FUNCTION p11_logicnaFunkcija : BOOL
VAR_INPUT
	x1: BOOL;
	x2: BOOL;
END_VAR
VAR_OUTPUT
	y: BOOL;
END_VAR
VAR // added by the converter: edge detectors and wires of the graphical bodies
    _w1 : BOOL;
END_VAR

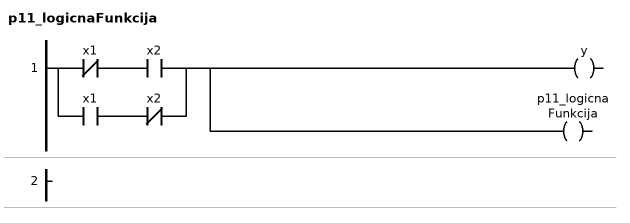
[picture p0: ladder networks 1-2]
// NETWORK 1
_w1 := NOT x1 AND x2 OR x1 AND NOT x2;
y := _w1;
p11_logicnaFunkcija := _w1;

// NETWORK 2

END_FUNCTION
